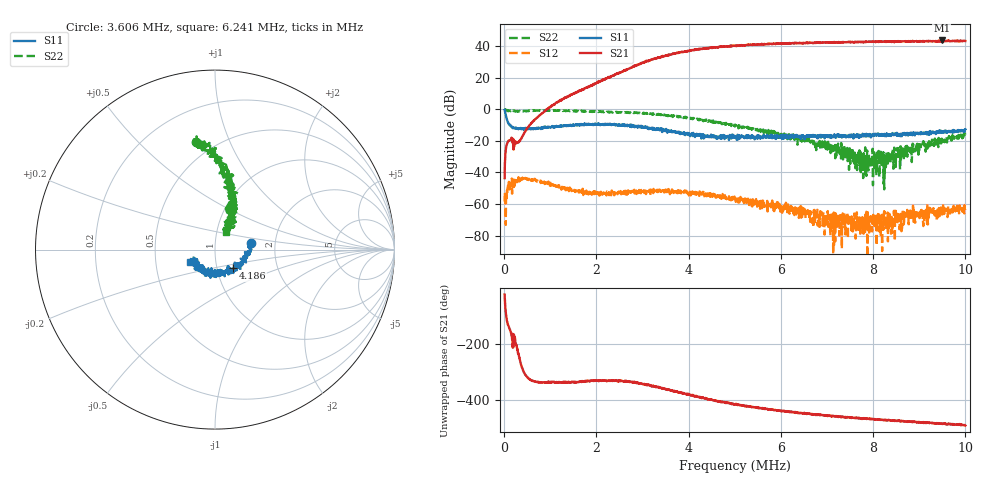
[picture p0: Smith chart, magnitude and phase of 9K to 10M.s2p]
!Keysight Technologies,P5004A,MY58100454,A.19.30.04
!Date: Wednesday, May 21, 2025 09:25:46
!Correction: S11(C  2-Port  )
!S21(C  2-Port  )
!S12(C  2-Port  )
!S22(C  2-Port  )
!S2P File: Measurements: S11, S21, S12, S22:
# Hz S  dB  R 50
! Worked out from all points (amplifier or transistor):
!   1601 points, 9 kHz to 10 MHz, reference 50 ohm
!   highest |S21| = 43.4 dB at 9.488 MHz (marker M1)
!   |S21| within 3 dB of that: 5.228 MHz to end of sweep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
!   unconditionally stable (mu >= 1): start of sweep to end of sweep
!   at 1.67 MHz: K = 8.90, MAG = 19.3 dB, |S12| = -51.4 dB
!   at 5.005 MHz: K = 2.83, MAG = 40.5 dB, |S12| = -55.7 dB
!   at 10 MHz: K = 4.99, MAG = 43.4 dB, |S12| = -63.6 dB
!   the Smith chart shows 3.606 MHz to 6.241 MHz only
!   S11 on the Smith chart (normalised r, x): 3.606 MHz: 1.50, +0.12; 4.186 MHz: 1.20, -0.26; 6.241 MHz: 0.75, -0.10
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9000  -0.55 -21.2  -43.57 -25.8  -58.42 93.4  -0.19 -19.2
1676248  -9.75 143.4  12.15 23.9  -52.70 -50.9  -1.20 152.1
2537972  -10.51 93.8  23.37 28.2  -53.81 -32.2  -2.07 131.2
3000056  -11.36 61.9  29.15 16.9  -50.93 -48.8  -2.71 116.7
3343496  -12.07 33.3  32.69 7.1  -52.51 -59.0  -2.97 108.6
3605760  -13.70 10.5  34.38 -4.5  -51.45 -73.2  -4.31 100.1
3805580  -14.70 -14.1  35.70 -12.8  -53.30 -74.4  -4.67 96.1
4186487  -16.72 -45.7  37.69 -27.6  -53.06 -88.2  -6.09 86.0
4511194  -17.02 -69.6  38.65 -38.5  -55.28 -98.6  -8.43 81.8
4698526  -16.78 -80.9  39.66 -45.2  -56.06 -85.3  -8.86 76.3
5004500  -16.93 -104.4  40.08 -55.7  -55.72 -106.2  -10.88 69.5
5316719  -16.96 -121.7  40.64 -62.4  -57.95 -106.9  -12.54 64.6
5610204  -18.30 -135.8  41.11 -69.3  -57.73 -123.5  -12.96 62.9
6240886  -16.28 -153.8  41.58 -81.9  -61.70 -113.7  -18.85 57.7
6671748  -16.49 -162.2  41.93 -89.9  -67.91 -131.9  -20.52 57.8
7083877  -16.47 -171.4  42.22 -94.5  -66.64 -118.6  -21.77 39.1
8338996  -16.76 176.7  42.86 -109.5  -71.32 -48.9  -32.08 -44.1
8420173  -15.10 167.9  42.65 -113.0  -73.28 -71.1  -25.02 -68.2
8900990  -16.61 160.2  42.92 -116.3  -68.00 -93.8  -24.85 -72.8
9487961  -14.97 156.4  43.42 -123.8  -63.91 -50.9  -18.63 -98.5
9887601  -14.15 155.6  42.94 -127.0  -62.86 -76.3  -17.35 -94.5
1e7  -12.75 145.6  43.06 -129.6  -63.63 -65.6  -16.13 -98.2
